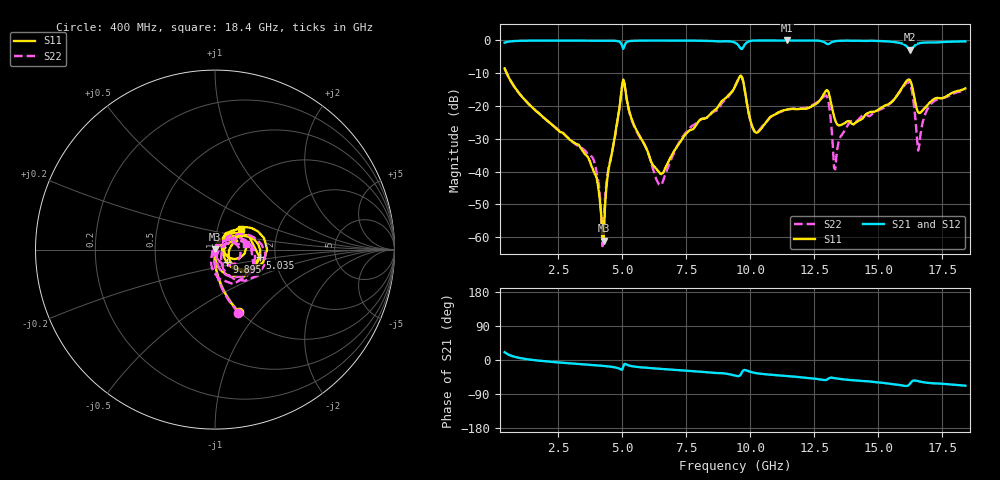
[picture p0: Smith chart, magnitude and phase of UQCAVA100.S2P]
!  Part Number  UQCAVA100	Mounting Orientation: Horizontal
!  Description: RF capacitors
!  Application: Coupling, Bypass, Tuning, DC Block
!  Filters, Matching
# GHZ S DB R 50
! Freq  |S11|  S11 Ph  |S21|  S21 Ph  |S12|  S12 Ph  |S22|  S22 Ph
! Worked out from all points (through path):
!   401 points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, 400 MHz to 18.4 GHz, reference 50 ohm
!   highest |S21| = -0.01 dB at 11.43 GHz (marker M1); lowest = -2.8 dB at 16.24 GHz (marker M2)
!   group delay of S21, straight-line fit = 11.3 ps
!   lowest |S11| = -61.0 dB at 4.27 GHz (marker M3), VSWR 1.00, Z = 50 + j0.0853 ohm
!   |S11| at or under -10 dB: 482.3 MHz to end of sweep
!   |S22| runs from -62.7 to -8.5 dB; largest |S21 - S12| = 0.0021
!   S11 on the Smith chart (normalised r, x): 400 MHz: 0.99, -0.80; 5.035 GHz: 1.65, -0.16; 9.895 GHz: 1.13, -0.16; 18.4 GHz: 1.29, +0.31
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0.4  -8.53 -69.0  -0.67 20.6  -0.67 20.6  -8.54 -69.5
3.415  -33.27 -104.5  -0.05 -11.1  -0.05 -11.1  -32.80 -93.7
3.91  -40.51 -108.0  -0.06 -13.7  -0.06 -13.7  -37.24 -110.5
4.27  -61.04 105.8  -0.06 -15.7  -0.06 -15.7  -56.09 44.0
4.45  -39.76 74.0  -0.06 -16.9  -0.06 -16.9  -39.35 49.6
5.035  -11.95 -10.0  -2.57 -18.4  -2.57 -18.3  -12.06 -28.5
6.43  -40.17 -35.9  -0.05 -23.1  -0.05 -23.1  -43.90 172.3
7.375  -29.65 46.4  -0.07 -27.6  -0.07 -27.6  -29.18 62.6
9.4  -14.09 38.9  -0.68 -41.1  -0.68 -41.1  -13.91 24.1
9.67  -11.13 -14.6  -2.61 -32.6  -2.61 -32.6  -11.16 -31.9
9.895  -20.47 -47.0  -0.47 -28.6  -0.47 -28.6  -20.58 -65.9
10.255  -28.14 10.1  -0.03 -35.1  -0.03 -35.1  -28.09 -8.5
11.425  -21.07 45.5  -0.01 -42.1  -0.01 -42.1  -21.10 25.3
12.415  -20.05 41.8  -0.01 -48.6  0.00 -48.6  -19.76 22.8
13  -15.17 3.5  -1.08 -51.4  -1.08 -51.4  -17.20 -32.9
13.315  -24.35 -21.8  -0.22 -48.1  -0.23 -48.1  -39.33 11.8
13.9  -24.86 9.4  -0.10 -53.0  -0.10 -53.0  -24.82 48.5
15.43  -19.26 26.6  -0.34 -62.5  -0.34 -62.4  -19.43 34.2
16.24  -12.20 -18.5  -2.77 -62.4  -2.76 -62.4  -13.31 -41.9
16.6  -22.14 -10.3  -0.85 -56.6  -0.85 -56.6  -31.83 6.1
17.095  -18.35 21.9  -0.62 -61.2  -0.63 -61.2  -19.04 21.7
18.4  -14.63 39.1  -0.28 -67.8  -0.29 -67.7  -15.18 11.0
